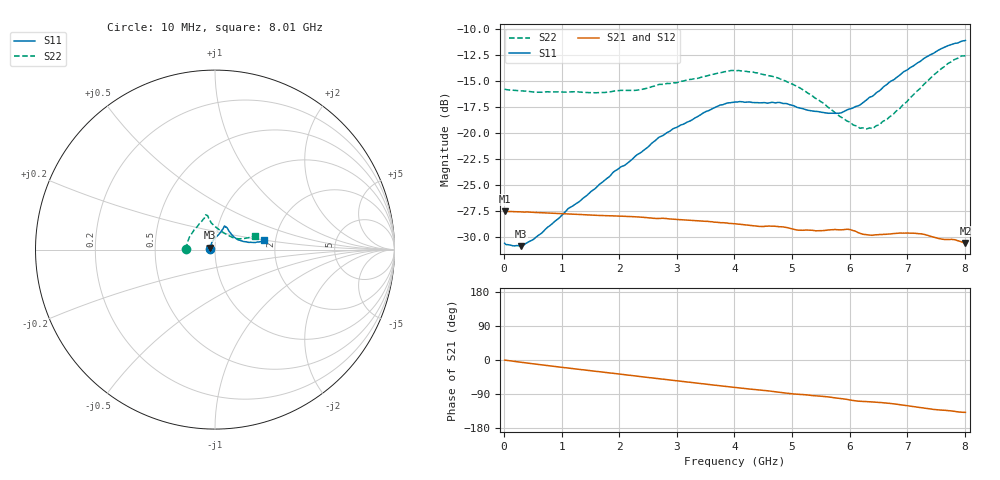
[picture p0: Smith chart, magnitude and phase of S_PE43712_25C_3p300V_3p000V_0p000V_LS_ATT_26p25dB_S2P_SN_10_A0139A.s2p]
! DEVICE ID: PE43712
! File Path: z:\PE43713\PE43713_CHAR_NOM_04292014\AMB\3p300\LS_ATT_26p25dB\PE43713_AMB_3p300V_3p000V_0p000V_LS_ATT_26p25dB_S2P_SN_10_A0139A.s2p
! Serial: 10
! Lot: A0139A
! Temp: 25C
! VDD: 3.300
! VSS: 0.000
! Control_Hi: 3.000
! Control_Lo: 0.000
! Attenuation Step: 26.25dB
! Port 1: RF1
! Port 2: RF2
! ThroughPath:1-2
! IDD: 0.0001451352
! ISS: -8.22e-008
#  Hz  S  RI  R  50
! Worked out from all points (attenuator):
!   801 points, 10 MHz to 8.01 GHz, reference 50 ohm
!   highest |S21| = -27.51 dB at 20 MHz (marker M1); lowest = -30.6 dB at 8.01 GHz (marker M2)
!   lowest |S11| = -30.9 dB at 290 MHz (marker M3), VSWR 1.06, Z = 47.4 + j1.03 ohm
!   |S11| at or under -10 dB: start of sweep to end of sweep
!   |S22| runs from -19.6 to -12.5 dB; largest |S21 - S12| = 0.00016
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1e7  -0.0296 0.000785  0.0421 -0.000184  0.0421 -0.000189  -0.163 0.00111
2e7  -0.0293 0.00139  0.0421 -0.000336  0.0421 -0.000317  -0.1627 0.00204
2.9e8  -0.0265 0.0109  0.0417 -0.00426  0.0417 -0.00425  -0.1589 0.0184
6.3e8  -0.0236 0.0227  0.0405 -0.00887  0.0405 -0.00888  -0.1531 0.038
1.12e9  -0.0179 0.0397  0.038 -0.0149  0.0381 -0.0149  -0.1439 0.0658
1.35e9  -0.0133 0.0462  0.0367 -0.0175  0.0367 -0.0175  -0.1376 0.0769
2.28e9  0.013 0.0765  0.0294 -0.0266  0.0294 -0.0266  -0.1019 0.1247
2.68e9  0.0267 0.0915  0.0255 -0.0294  0.0255 -0.0294  -0.0832 0.1501
3.5e9  0.0457 0.1186  0.0168 -0.0338  0.0167 -0.0338  -0.0574 0.1793
3.74e9  0.0496 0.1271  0.014 -0.0344  0.014 -0.0344  -0.0543 0.1881
4.01e9  0.0534 0.131  0.0111 -0.035  0.0111 -0.035  -0.0526 0.1937
4.76e9  0.0637 0.1256  0.00323 -0.0354  0.00327 -0.0354  -0.037 0.1808
5.35e9  0.0803 0.0998  -0.00219 -0.0341  -0.00219 -0.0341  -0.0217 0.1502
5.82e9  0.1012 0.0735  -0.00671 -0.0337  -0.0067 -0.0337  0.00977 0.1208
5.99e9  0.113 0.0657  -0.00898 -0.0333  -0.0089 -0.0333  0.0248 0.1109
6.18e9  0.1249 0.0562  -0.0107 -0.0312  -0.0107 -0.0312  0.0435 0.0965
6.4e9  0.1425 0.0503  -0.0113 -0.0303  -0.0113 -0.0303  0.0668 0.0818
6.68e9  0.1699 0.0436  -0.0135 -0.0298  -0.0134 -0.0298  0.0982 0.0673
7.15e9  0.2119 0.0396  -0.0183 -0.0274  -0.0183 -0.0274  0.1457 0.0607
7.56e9  0.2492 0.0436  -0.0207 -0.0232  -0.0207 -0.0232  0.19 0.0675
7.81e9  0.2659 0.0481  -0.0219 -0.0216  -0.0219 -0.0216  0.2131 0.0744
8.01e9  0.275 0.0522  -0.0221 -0.0198  -0.022 -0.0198  0.224 0.0764
